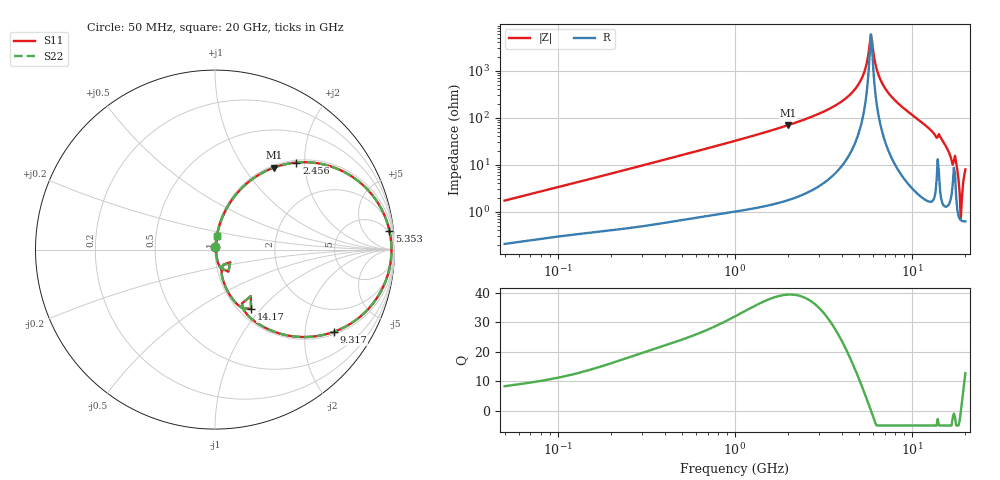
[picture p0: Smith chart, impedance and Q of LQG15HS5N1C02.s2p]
!Murata Part Number: LQG15HS5N1C02
!These Parameters are Measured in Series Mode Connection
!  o--[Z]--o
!Port1  Port2
!  o-------o
!Freq. Start=50[MHz] Stop=20[GHz], 401[Steps]
# Hz S RI R 50
!Freq.(Hz) S11(Real) S11(Imag) S21(Real) S21(Imag) S12(Real) S12(Imag) S22(Real) S22(Imag)
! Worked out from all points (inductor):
!   401 points, 50 MHz to 20 GHz, reference 50 ohm
!   read as one part in series: L = 5.39 nH near 51.52 MHz
!   highest Q = 39.3 at 1.992 GHz (marker M1), where L = 5.53 nH
!   self-resonance near 5.856 GHz
!   S11 on the Smith chart (normalised r, x): 50 MHz: 1.00, +0.03; 2.456 GHz: 1.05, +1.82; 5.353 GHz: 4, +18; 9.317 GHz: 1.09, -2.83; 14.17 GHz: 1.14, -0.88; 20 GHz: 1.01, +0.16
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5e7  0.00236 0.0171  0.9976 -0.0171  0.9976 -0.0171  0.00236 0.0171
1.364002e8  0.00537 0.0443  0.9946 -0.0443  0.9946 -0.0443  0.00537 0.0443
3.721004e8  0.0193 0.1162  0.9807 -0.1162  0.9807 -0.1162  0.0193 0.1162
1e9  0.1009 0.286  0.8991 -0.286  0.8991 -0.286  0.1009 0.286
1.99176e9  0.3278 0.4569  0.6722 -0.4569  0.6722 -0.4569  0.3278 0.4569
2.456456e9  0.4536 0.485  0.5464 -0.485  0.5464 -0.485  0.4536 0.485
2.728004e9  0.5271 0.4859  0.4729 -0.4859  0.4729 -0.4859  0.5271 0.4859
4.275624e9  0.8659 0.3171  0.1341 -0.3171  0.1341 -0.3171  0.8659 0.3171
4.89267e9  0.9408 0.199  0.0592 -0.199  0.0592 -0.199  0.9408 0.199
5.352748e9  0.9719 0.1047  0.0281 -0.1047  0.0281 -0.1047  0.9719 0.1047
5.856089e9  0.9834 0.00154  0.0166 -0.00154  0.0166 -0.00154  0.9834 0.00154
6.034176e9  0.9822 -0.0341  0.0178 0.0341  0.0178 0.0341  0.9822 -0.0341
6.503449e9  0.9674 -0.1238  0.0326 0.1238  0.0326 0.1238  0.9674 -0.1238
7.442007e9  0.8963 -0.278  0.1037 0.278  0.1037 0.278  0.8963 -0.278
9.316812e9  0.6618 -0.4582  0.3382 0.4582  0.3382 0.4582  0.6618 -0.4582
1.149051e10  0.3729 -0.471  0.6271 0.471  0.6271 0.471  0.3729 -0.471
1.417136e10  0.201 -0.3299  0.799 0.3299  0.799 0.3299  0.201 -0.3299
1.774144e10  0.0311 -0.1032  0.9689 0.1032  0.9689 0.1032  0.0311 -0.1032
1.828096e10  0.0104 -0.0478  0.9896 0.0478  0.9896 0.0478  0.0104 -0.0478
1.88369e10  0.00658 -0.00247  0.9934 0.00247  0.9934 0.00247  0.00658 -0.00247
1.940974e10  0.00776 0.0388  0.9922 -0.0388  0.9922 -0.0388  0.00776 0.0388
2e10  0.0123 0.0777  0.9877 -0.0777  0.9877 -0.0777  0.0123 0.0777
